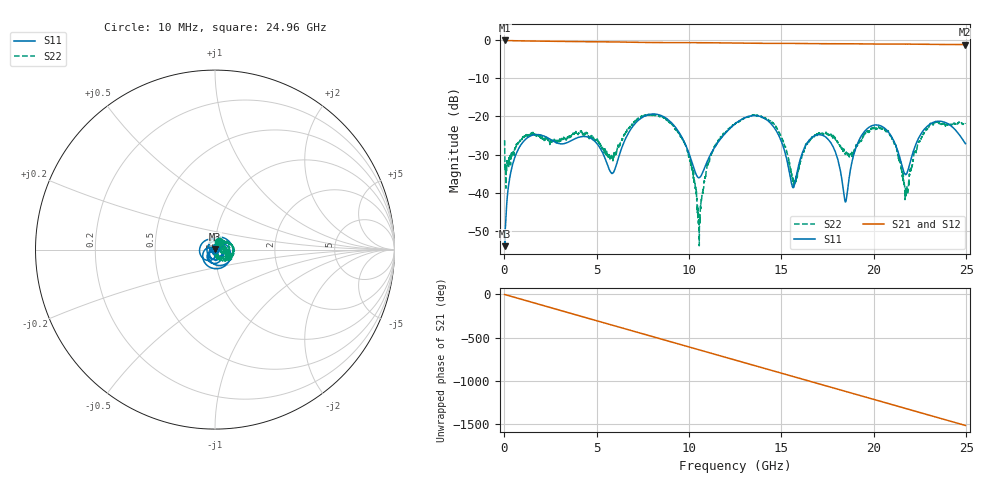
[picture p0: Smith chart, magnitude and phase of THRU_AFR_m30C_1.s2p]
!Keysight Technologies,M9372A,MY54321388,A.12.55.09
!Automatic Fixture Removal (AFR)
!Date: Wednesday, May 22, 2019 8:35:12 AM
!S2P File: Measurements: S11,S21,S12,S22:
# MHz S  RI  R 50
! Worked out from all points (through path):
!   2496 points, 10 MHz to 24.96 GHz, reference 50 ohm
!   highest |S21| = -0.01 dB at 40 MHz (marker M1); lowest = -1.1 dB at 24.92 GHz (marker M2)
!   group delay of S21, straight-line fit = 168 ps
!   lowest |S11| = -54.1 dB at 20 MHz (marker M3), VSWR 1.00, Z = 50 + j0.191 ohm
!   |S11| at or under -10 dB: start of sweep to end of sweep
!   |S22| runs from -54.0 to -19.4 dB; largest |S21 - S12| = 1.5e-15
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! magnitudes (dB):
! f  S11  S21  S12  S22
! 10 MHz  -51.7  -0.1  -0.1  -26.2
! 20 MHz  -54.1  0.0  0.0  -30.8
! 40 MHz  -50.9  0.0  0.0  -34.1
! 1.03 GHz  -26.6  -0.1  -0.1  -25.2
! 4.17 GHz  -25.3  -0.3  -0.3  -23.8
! 5.85 GHz  -34.9  -0.4  -0.4  -30.9
! 8.33 GHz  -19.5  -0.6  -0.6  -19.9
! 9.75 GHz  -26.8  -0.6  -0.6  -27.1
! 10.53 GHz  -36.1  -0.6  -0.6  -49.8
! 11.24 GHz  -29.3  -0.6  -0.6  -29.6
! 12.49 GHz  -21.9  -0.7  -0.7  -21.9
! 14.41 GHz  -21.8  -0.8  -0.8  -21.2
! 15.63 GHz  -38.7  -0.8  -0.8  -36.9
! 16.65 GHz  -25.5  -0.8  -0.8  -25.4
! 17.73 GHz  -27.4  -0.9  -0.9  -25.0
! 18.47 GHz  -42.5  -0.9  -0.9  -29.7
! 19.38 GHz  -24.7  -0.9  -0.9  -25.7
! 20.81 GHz  -24.2  -1.0  -1.0  -24.3
! 21.78 GHz  -35.1  -1.0  -1.0  -39.4
! 22.98 GHz  -22.2  -1.0  -1.0  -22.7
! 24.92 GHz  -26.8  -1.1  -1.1  -21.9
! 24.96 GHz  -27.1  -1.1  -1.1  -21.9
